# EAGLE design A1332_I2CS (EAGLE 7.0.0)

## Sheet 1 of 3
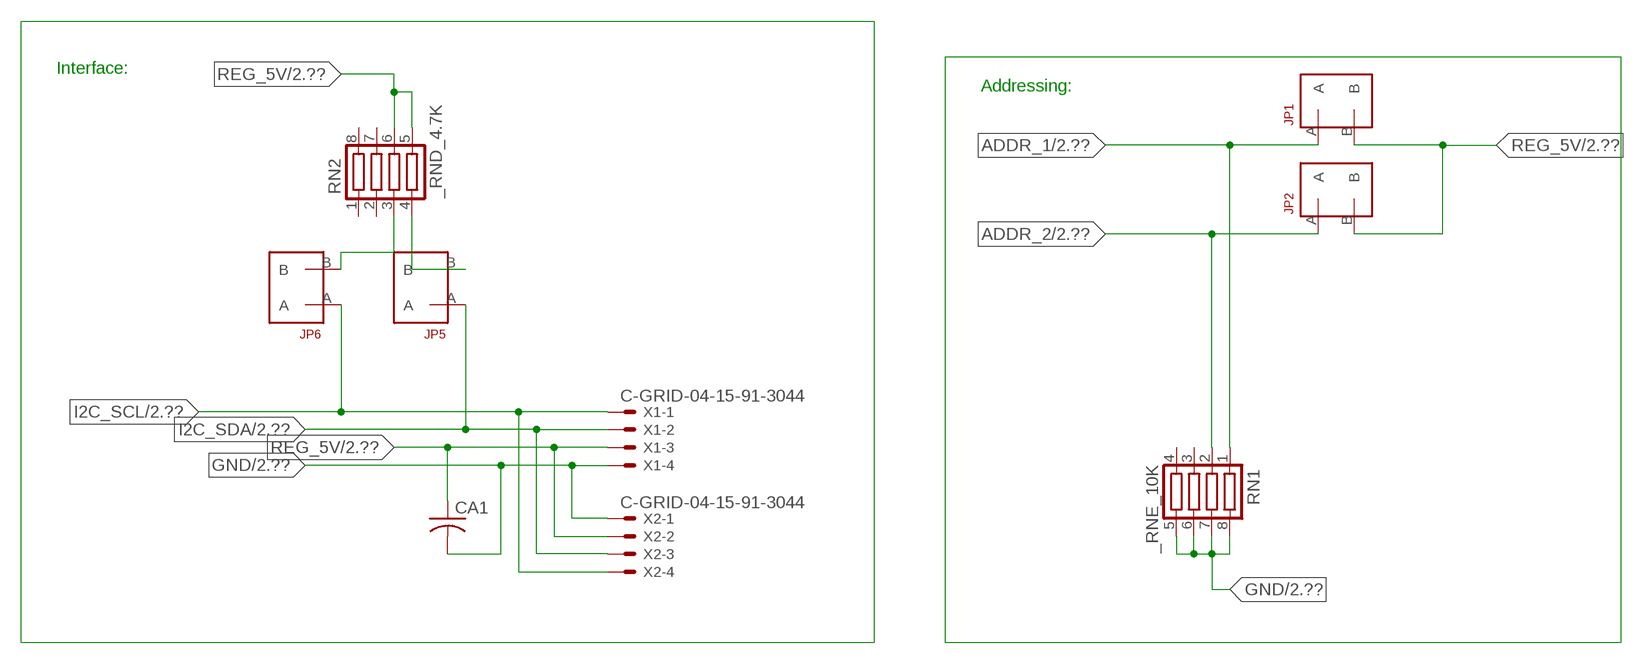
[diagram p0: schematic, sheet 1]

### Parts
CA1  CC1206KRX7R9BB104  [.1UF]
JP1  JUMPER_1X2_2MM  [JUMPER_1X2_2MM]
JP2  JUMPER_1X2_2MM  [JUMPER_1X2_2MM]
JP5  JUMPER_1X2_2MM  [JUMPER_1X2_2MM]
JP6  JUMPER_1X2_2MM  [JUMPER_1X2_2MM]
RN1  _RNE_10K  [RNE]
RN2  _RND_4.7K  [RND]
X1  C-GRID-04-15-91-3044  [15-91-04]
X2  C-GRID-04-15-91-3044  [15-91-04]

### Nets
ADDR_1: JP1.A RN1.1 ; also sheet 2
ADDR_2: JP2.A RN1.2 ; also sheet 2
GND: CA1.2 RN1.5 RN1.6 RN1.7 RN1.8 X1.4 X2.1 ; also sheet 2,3
I2C_SCL: JP6.A X1.1 X2.4 ; also sheet 2
I2C_SDA: JP5.A X1.2 X2.3 ; also sheet 2
N$1: JP6.B RN2.3
N$2: JP5.B RN2.4
REG_5V: CA1.1 JP1.B JP2.B RN2.5 RN2.6 X1.3 X2.2 ; also sheet 2,3
Unconnected: RN1.3 RN1.4 RN2.1 RN2.2 RN2.7 RN2.8

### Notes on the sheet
- Interface:
- Addressing:

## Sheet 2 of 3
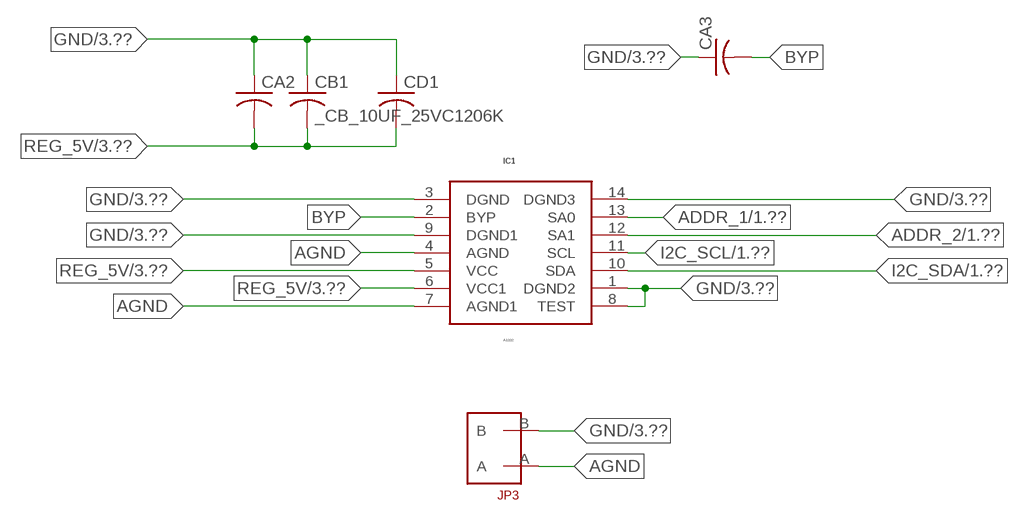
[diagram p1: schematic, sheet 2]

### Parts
CA2  _CA_.10UF_50VC1206K  [_CA_.1UF_50V]
CA3  _CA_.10UF_50VC1206K  [_CA_.1UF_50V]
CB1  _CB_10UF_25VC1206K  [_CB_10UF_25V]
CD1  _CD_10NF_50VC1206K  [_CD_10NF_50V]
IC1  A1332  [TSSOP-14]
JP3  JUMPER_1X2_2MM  [JUMPER_1X2_2MM]

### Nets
ADDR_1: IC1.13(SA0) ; also sheet 1
ADDR_2: IC1.12(SA1) ; also sheet 1
AGND: IC1.4(AGND) IC1.7(AGND1) JP3.A
BYP: CA3.2 IC1.2(BYP)
GND: CA2.1 CA3.1 CB1.1 CD1.1 IC1.1(DGND2) IC1.3(DGND) IC1.8(TEST) IC1.9(DGND1) IC1.14(DGND3) JP3.B ; also sheet 1,3
I2C_SCL: IC1.11(SCL) ; also sheet 1
I2C_SDA: IC1.10(SDA) ; also sheet 1
REG_5V: CA2.2 CB1.2 CD1.2 IC1.5(VCC) IC1.6(VCC1) ; also sheet 1,3

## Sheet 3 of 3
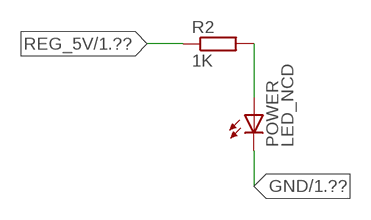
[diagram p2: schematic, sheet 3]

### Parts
POWER  LED_NCD  [CHIPLED_0603]
R2  1K  RESISTOR_SMT-0402  [R402]

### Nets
GND: POWER.C ; also sheet 1,2
N$13: POWER.A R2.2
REG_5V: R2.1 ; also sheet 1,2

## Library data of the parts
CA1 = NCD_ULTIMATE_LIBRARY:CC1206KRX7R9BB104: Capacitor CA .1uF 50V SMT C1206K CC1206KRX7R9BB104
CA2 CA3 = NCD_ULTIMATE_LIBRARY:_CA_.10UF_50V: Capacitor .1uF SMT
CB1 = NCD_ULTIMATE_LIBRARY:_CB_10UF_25V: Capacitor 10uF SMT
CD1 = NCD_ULTIMATE_LIBRARY:_CD_10NF_50V: Capacitor 10nF SMT
IC1 = NCD_ULTIMATE_bhaskar:A1332: Digikey 620-1687-2-ND/A1332ELETR-T
JP1-JP3 JP5 JP6 = NCD_ULTIMATE_CONNECTORS:JUMPER_1X2_2MM
POWER = NCD_ULTIMATE_LIBRARY:LED_NCD: LED Digikey 754-1132-2-ND/APT2012SRCPRV
R2 = NCD_ULTIMATE_LIBRARY:RESISTOR_SMT: NCD Resistor
RN1 = NCD_ULTIMATE_LIBRARY:_RNE_10K: Resistor Array RNE SMT 10K x 4 Single Resistor Source: http://www.ctscorp.com/components/Datasheets/CTSChipArrayDs.pdf Digikey 742C083103JPTR-ND/742C083103JP; OC_FARNELL: unknown; OC_NEWARK: unknown
RN2 = NCD_ULTIMATE_LIBRARY:_RND_4.7K: Resistor Array RND SMT 4.7K x 4 Single Resistor Source: http://www.ctscorp.com/components/Datasheets/CTSChipArrayDs.pdf Digikey 742C083472JPTR-ND/742C083472JP; OC_FARNELL: unknown; OC_NEWARK: unknown
X1 X2 = NCD_ULTIMATE_CONNECTORS:C-GRID-04: CONNECTOR 4-Pos I2C wire to board 2.54 mm (0.100") pitch header Digikey WM1342-ND/0015912045; OC_FARNELL: unknown; OC_NEWARK: unknown

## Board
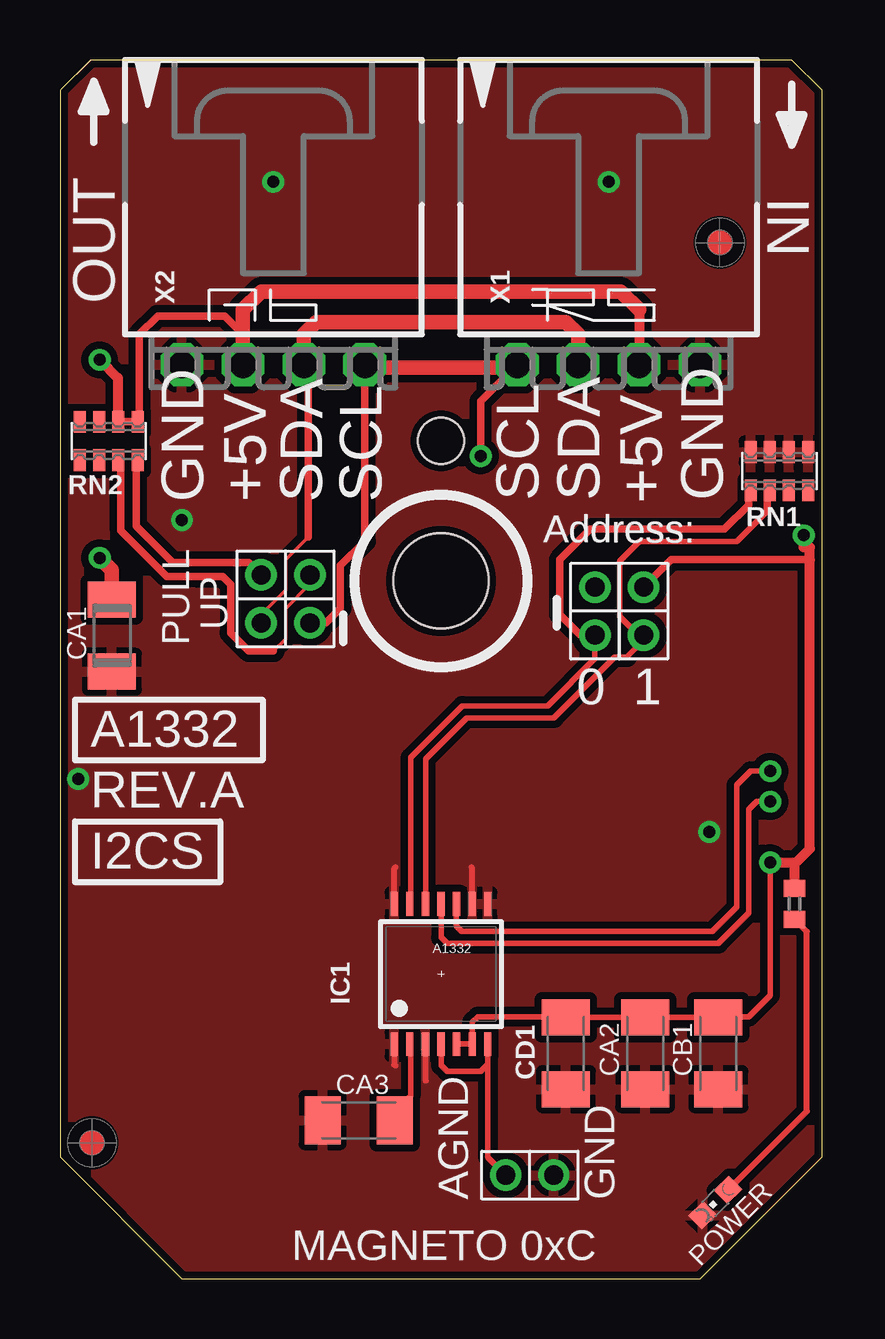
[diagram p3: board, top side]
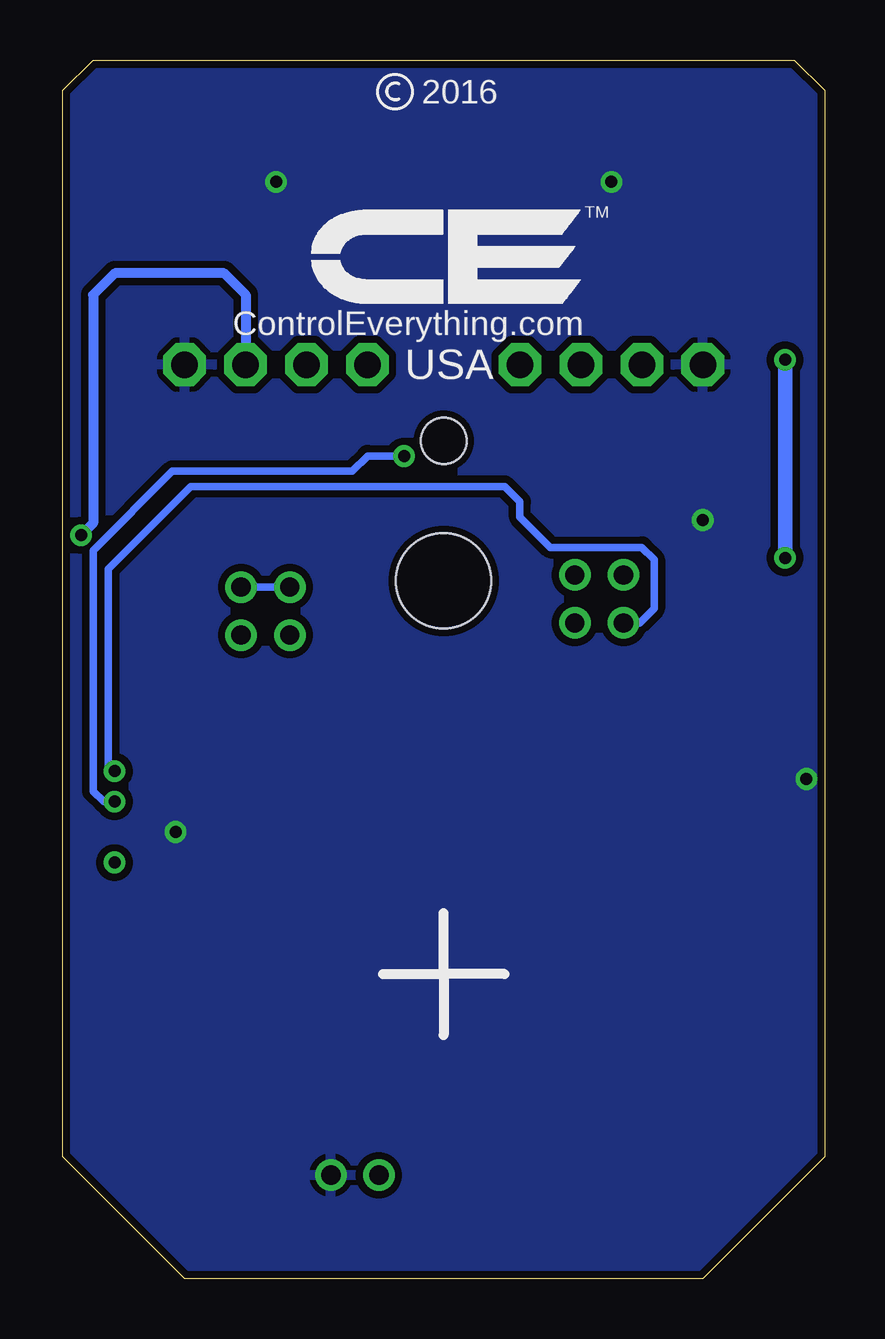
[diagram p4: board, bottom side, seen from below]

Size 31.75 x 50.8 mm. Coordinates in mm from the lower left corner, seen from the top.
Outline: 32 segments
Copper layers (1*16): Top 0.035mm / dielectric 1.5mm / Bottom 0.035mm
Design rules "default": minimum track width 5mil, minimum drill 24mil, track to track 5mil, track to pad 5mil, pad to pad 5mil, via to via 5mil, smd to smd 5mil, copper to edge 10mil, drill to drill 8mil, minimum pad ring 10mil, minimum via ring 8mil, stop-mask expansion 2mil, vias tented up to drill 0mil, thermal gap 10mil
Holes 3.96 mm at 15.88,29.08
Holes 1.91 mm at 15.88,34.92

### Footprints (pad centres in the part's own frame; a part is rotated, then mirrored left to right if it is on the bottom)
.1UF = smd 1.5 x 2: 1 -1.5,0; 2 1.5,0
_CA_.1UF_50V = smd 1.5 x 2: 1 -1.5,0; 2 1.5,0
_CB_10UF_25V = smd 1.5 x 2: 1 -1.5,0; 2 1.5,0
_CD_10NF_50V = smd 1.5 x 2: 1 -1.5,0; 2 1.5,0
TSSOP-14 = smd 0.305 x 0.991: 1 -1.95,-2.918; 2 -1.3,-2.918; 3 -0.65,-2.918; 4 0,-2.918; 5 0.65,-2.918; 6 1.3,-2.918; 7 1.95,-2.918; 8 1.95,2.918; 9 1.3,2.918; 10 0.65,2.918; 11 0,2.918; 12 -0.65,2.918; 13 -1.3,2.918; 14 -1.95,2.918
JUMPER_1X2_2MM = drill 0.8: A 0,2; B 0,0
CHIPLED_0603 = smd 0.8 x 0.876: A 0,-0.75; C 0,0.75
R402 = smd 0.7 x 0.9: 1 -0.65,0; 2 0.65,0
RNE = smd 0.5 x 0.9: 1 -1.2,-0.8; 2 -0.4,-0.8; 3 0.4,-0.8; 4 1.2,-0.8; 5 1.2,0.8; 6 0.4,0.8; 7 -0.4,0.8; 8 -1.2,0.8
RND = smd 0.5 x 0.9: 1 -1.2,-0.8; 2 -0.4,-0.8; 3 0.4,-0.8; 4 1.2,-0.8; 5 1.2,0.8; 6 0.4,0.8; 7 -0.4,0.8; 8 -1.2,0.8
15-91-04 = drill 1.1 pad 1.778 octagon: 1 -3.81,-7.62; 2 -1.27,-7.62; 3 1.27,-7.62; 4 3.81,-7.62

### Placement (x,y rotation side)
CA1  2.16,26.81 270 top
CA2  24.38,9.4 90 top
CA3  12.45,6.6 0 top
CB1  27.43,9.4 90 top
CD1  21.08,9.4 90 top
IC1  15.88,12.7 0 top
JP1  22.29,28.83 180 top
JP2  24.32,28.83 180 top
JP3  20.57,4.32 90 top
JP5  8.38,29.34 180 top
JP6  10.41,29.34 180 top
POWER  27.3,3.18 135 top
R2  30.61,15.62 270 top
RN1  29.97,33.66 0 top
RN2  2.03,34.92 0 top
U$5  [VISION_REF10]  1.33,5.66 90 top
U$28  [VISION_REF10]  27.5,43.19 90 top
X1  22.86,45.72 0 top
X2  8.89,45.72 0 top

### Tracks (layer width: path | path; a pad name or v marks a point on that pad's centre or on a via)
ADDR_1
  Top 0.229: IC1.13 14.61,15.78 14.61,21.72 16.76,23.88 20.32,23.88 22.29,25.85 JP1.A
  Top 0.305: RN1.1 28.7,32.79 28.7,32.26 27.69,31.24 22.1,31.24 20.83,29.97 20.83,27.69 21.68,26.83 JP1.A
ADDR_2
  Top 0.229: IC1.12 15.24,15.63 15.24,21.67 16.94,23.37 20.57,23.37 23.11,25.91 23.62,25.91 24.32,26.61 JP2.A 24.1,26.83 23.32,27.61 23.32,29.92 24.13,30.73 28.19,30.73 29.46,32
  Top 0.305: RN1.2 29.46,32.75 29.46,32
AGND
  Top 0.229: IC1.4 15.88,8.89 16.13,8.64 17.53,8.64 17.82,8.94 IC1.7 17.83,8.76 17.83,5.06 JP3.A
BYP
  Top 0.229: IC1.2 14.61,9.37 14.61,7.62 13.95,7.09 CA3.2
GND  (via drill 0.5)
  Top 0.254: IC1.9 17.18,17.12 17.14,17.15 | IC1.14 13.93,17.1 13.97,17.15 | IC1.3 15.22,8.27 15.24,8.26 | IC1.1 13.93,8.94 13.97,8.89
  other vias: 8.89,45.72 22.86,45.72 27.05,18.62 0.76,20.83 5.08,31.62
  pour Bottom (isolate 0.305): 4.45,-0.63 -0.64,4.45 -0.64,50.17 0.64,51.44 31.11,51.44 32.38,50.17 32.38,4.45 27.3,-0.63
  pour Top (isolate 0.305): 3.81,-1.27 -1.27,3.81 -1.27,50.8 0,52.07 31.75,52.07 33.02,50.8 33.02,3.81 27.94,-1.27
I2C_SCL  (via drill 0.5)
  Top 0.229: IC1.11 15.88,14.22 16.13,13.97 27.43,13.97 28.7,15.24 28.7,19.56 29.03,19.89 v29.59,19.89
  Top 0.305: 12.7,37.97 12.7,30.73 11.68,29.72 11.68,27.94 11.08,27.34 JP6.A | v17.53,34.29 17.53,36.58 X1.1
  Top 0.406: X2.4 12.7,37.97 | 19.05,37.97 X1.1
  Top 0.61: 12.7,37.97 19.05,37.97
  Bottom 0.305: v29.59,19.89 30.05,19.89 30.48,20.32 30.48,30.35 27.18,33.66 19.68,33.66 19.05,34.29 v17.53,34.29
I2C_SDA  (via drill 0.5)
  Top 0.152: 10.35,30.92 9.4,29.97 9.4,28.7 8.38,27.69 JP5.A
  Top 0.229: IC1.10 16.51,15.22 16.51,14.71 16.74,14.48 27.18,14.48 28.19,15.49 28.19,20.57 28.78,21.16 v29.59,21.16
  Top 0.305: 10.35,30.92 10.35,37.91 X2.3
  Top 0.61: X2.3 10.16,39.37 10.67,39.88 21.08,39.88 21.59,39.37 X1.2
  Bottom 0.305: v29.59,21.16 29.84,21.41 29.84,29.59 26.42,33.02 13.34,33.02 12.7,32.39 12.7,31.75 11.43,30.48 7.62,30.48 7.11,29.97 7.11,27.94 7.71,27.34 JP5.A
N$1
  Top 0.152: 8.89,26.16 9.4,26.67 9.4,27.94 10.41,28.96 JP6.B
  Top 0.305: RN2.3 2.54,34.02 2.54,31.18 4.45,29.27 5.75,29.27 5.76,29.26 6.78,29.26 7.11,28.93 7.11,26.92 7.87,26.16 8.89,26.16
N$2
  Top 0.305: RN2.4 3.17,34.07 3.17,31.37 4.7,29.85 6.1,29.85 6.35,29.85 7.87,29.85 JP5.B
N$13
  Top 0.254: POWER.A 31.11,6.99 31.11,14.46 R2.2
REG_5V  (via drill 0.5)
  Top 0.229: v29.59,17.35 29.59,11.81 28.7,10.92 27.46,10.92 CB1.2 CA2.2 CD1.2 21.06,10.92 17.4,10.92 17.18,10.7 IC1.6 IC1.5
  Top 0.305: 7.62,39.37 7.49,39.37 | RN2.6 RN2.5 3.3,35.8 3.3,39.37 4.06,40.13 6.86,40.13 7.62,39.37 | 7.62,40.39 7.62,39.37 | JP2.B 25.46,29.97 31.24,29.97
  Top 0.406: v29.59,17.35 30.67,17.35 | 30.67,17.35 31.24,17.92 31.24,29.97 31.24,30.48 30.99,30.48 v30.99,30.99 | v1.65,38.3 2.41,37.54 2.41,35.74 RN2.6 | R2.1 30.61,17.29 30.67,17.35 | 24.13,40.39 X1.3
  Top 0.61: X2.2 7.62,40.39 8.38,41.15 23.37,41.15 24.13,40.39 | CA1.1 2.16,29.54 v1.65,30.05
  Top 0.813: v30.99,30.99 31.05,30.99
  Bottom 0.305: JP1.B JP2.B
  Bottom 0.406: v30.99,30.99 30.48,31.5 30.48,41.01 29.58,41.91 25.03,41.91 24.13,41.01 X1.3
  Bottom 0.61: v1.65,30.05 v1.65,38.3

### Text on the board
tPlace: AGND | GND | MAGNETO 0xC
tNames: IN | OUT | GND | GND | +5V | +5V | SDA | SDA | SCL | SCL | SCL | SCL | SDA | SDA | +5V | +5V | GND | GND | Address: | Address: | UP | PULL | 0 | 1 | A1332 | REV.A | I2CS
bNames: 2016 | TM | ControlEverything.com | USA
